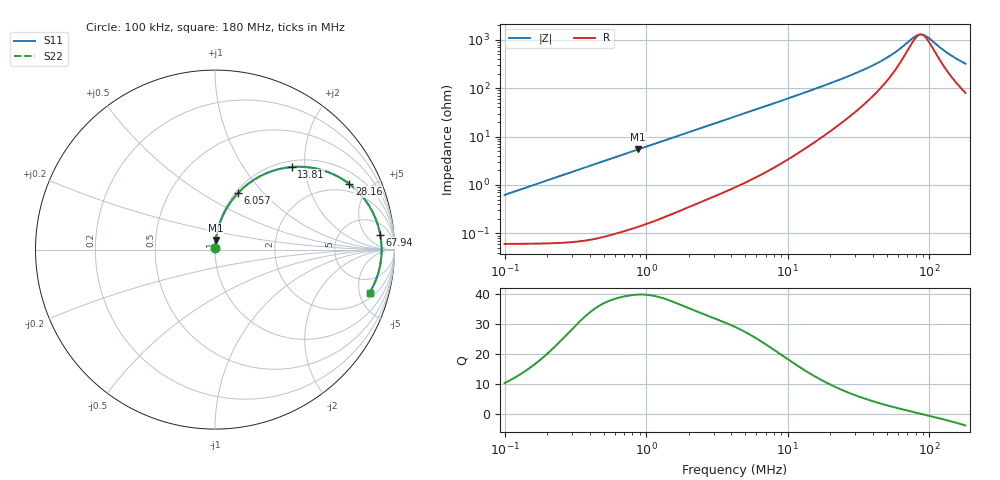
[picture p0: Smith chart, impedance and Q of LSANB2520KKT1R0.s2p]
! LSANB2520KKT1R0  S-PARAMETER MODEL  ( General Type )
! Model Generated by TAIYO YUDEN Corporation (http://www.ty-top.com)
! Version 2.0
! TAIYO YUDEN Control No. 20210629
! Copyright(c) 2013 TAIYO YUDEN CO.,LTD. All Rights Reserved.
! Product Description (link to TY-COMPAS)
! https://ds.yuden.co.jp/TYCOMPAS/or/detail?pn=LSANB2520KKT1R0M&u=M
! Products Name : Inductors
! Characteristics :
!  Inductance : 1.0 uH , SRF(min) : -Hz , DC Resistance(max) : 0.072 Ohm
!  Rated Current : Saturation :2700 mA , Temp Rise : 2500 mA (40 degC)
!  Case Size : 2.5 x 2.0 / 0.098 x 0.079 [mm/inch] , Thickness : 1 / 0.039 [mm/inch]
!  (Conditions: Temperature = 25 degC , DC Bias Current/Voltage = 0A / 0V)
! External Node Assignments :
!  1  o---GGG---o  2
! GND o---------o GND
! Frequency Range : 0.1MHz  -  180.004543MHz  [ 402 STEP ]
# MHz S RI R 50
! Freq[MHz].  S11 Real  S11 Imag  S21 Real  S21 Imag  S12 Real  S12 Imag  S22 Real  S22 Imag
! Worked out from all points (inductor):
!   401 points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, 100 kHz to 180 MHz, reference 50 ohm
!   read as one part in series: L = 987 nH near 103.8 kHz
!   highest Q = 39.9 at 879.1 kHz (marker M1), where L = 986 nH
!   self-resonance near 87.17 MHz
!   S11 on the Smith chart (normalised r, x): 100 kHz: 1.00, +0.01; 6.057 MHz: 1.03, +0.74; 13.81 MHz: 1.12, +1.70; 28.16 MHz: 1.56, +3.72; 67.94 MHz: 11, +13; 180 MHz: 2.61, -6.25
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0.1  0.000641 0.00619  0.9994 -0.00619  0.9994 -0.00619  0.000641 0.00619
0.350962  0.00117 0.0218  0.9988 -0.0218  0.9988 -0.0218  0.00117 0.0218
0.879088  0.00431 0.0541  0.9957 -0.0541  0.9957 -0.0541  0.00431 0.0541
1.231743  0.00766 0.0753  0.9923 -0.0753  0.9923 -0.0753  0.00766 0.0753
2.373325  0.0247 0.1412  0.9753 -0.1412  0.9753 -0.1412  0.0247 0.1412
4.322947  0.0722 0.242  0.9278 -0.242  0.9278 -0.242  0.0722 0.242
6.057141  0.1293 0.3162  0.8707 -0.3162  0.8707 -0.3162  0.1293 0.3162
8.977803  0.2422 0.4039  0.7578 -0.4039  0.7578 -0.4039  0.2422 0.4039
13.81494  0.4271 0.4601  0.5729 -0.4601  0.5729 -0.4601  0.4271 0.4601
14.89024  0.4635 0.4618  0.5365 -0.4618  0.5365 -0.4618  0.4635 0.4618
20.09616  0.6086 0.4393  0.3914 -0.4393  0.3914 -0.4393  0.6086 0.4393
28.15793  0.7487 0.3654  0.2513 -0.3654  0.2513 -0.3654  0.7487 0.3654
39.45378  0.8466 0.2621  0.1534 -0.2621  0.1534 -0.2621  0.8466 0.2621
52.25907  0.8962 0.1688  0.1038 -0.1688  0.1038 -0.1688  0.8962 0.1688
67.93547  0.9209 0.0818  0.0791 -0.0818  0.0791 -0.0818  0.9209 0.0818
80.41563  0.9275 0.0264  0.0725 -0.0264  0.0725 -0.0264  0.9275 0.0264
85.06583  0.9282 0.008  0.0718 -0.008  0.0718 -0.008  0.9282 0.008
89.98492  0.9282 -0.0104  0.0718 0.0104  0.0718 0.0104  0.9282 -0.0104
98.82363  0.9265 -0.0411  0.0735 0.0411  0.0735 0.0411  0.9265 -0.0411
138.4677  0.9026 -0.1526  0.0974 0.1526  0.0974 0.1526  0.9026 -0.1526
160.8623  0.8818 -0.2027  0.1182 0.2027  0.1182 0.2027  0.8818 -0.2027
180.0045  0.8615 -0.2401  0.1385 0.2401  0.1385 0.2401  0.8615 -0.2401
